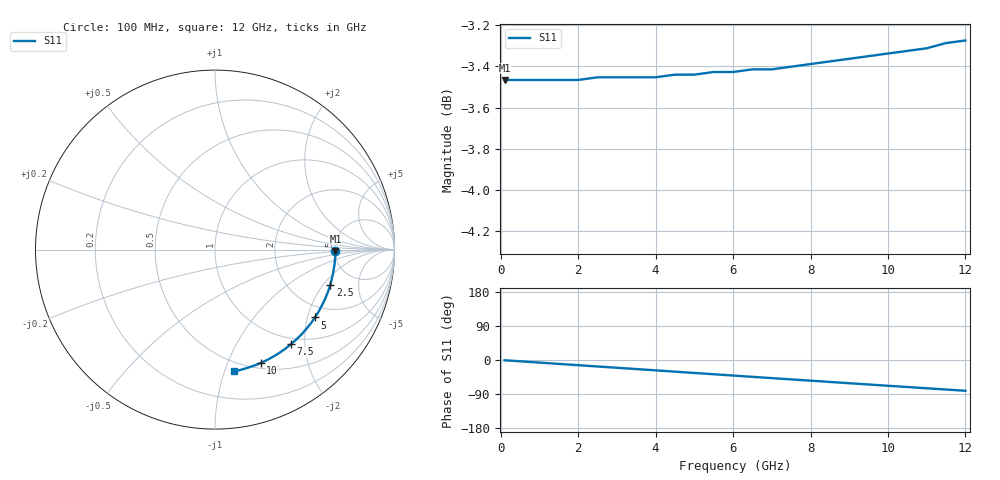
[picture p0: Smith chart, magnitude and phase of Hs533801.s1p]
!HSCH-5318 and HSCH-5338 Schottky diodes
!S-parameters at 1 mA self-bias.  Last updated 6/7/94
# ghz s ma r 50
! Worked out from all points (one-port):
!   25 points, 100 MHz to 12 GHz, reference 50 ohm
!   lowest |S11| = -3.5 dB at 100 MHz (marker M1), VSWR 5.08, Z = 254 - j7.57 ohm
!   |S11| at or under -10 dB: nowhere
!   S11 on the Smith chart (normalised r, x): 100 MHz: 5.07, -0.15; 2.5 GHz: 3.28, -2.37; 5 GHz: 1.61, -2.23; 7.5 GHz: 0.89, -1.73; 10 GHz: 0.56, -1.32; 12 GHz: 0.42, -1.08
0.1  0.671 -0.7
0.5  0.671 -3.4
1  0.671 -6.8
1.5  0.671 -10.3
2  0.671 -13.7
2.5  0.672 -17.1
3  0.672 -20.5
3.5  0.672 -23.9
4  0.672 -27.3
4.5  0.673 -30.8
5  0.673 -34.2
5.5  0.674 -37.6
6  0.674 -41.0
6.5  0.675 -44.4
7  0.675 -47.8
7.5  0.676 -51.2
8  0.677 -54.5
8.5  0.678 -57.9
9  0.679 -61.3
9.5  0.68 -64.6
10  0.681 -68.0
10.5  0.682 -71.3
11  0.683 -74.6
11.5  0.685 -77.9
12  0.686 -81.2
